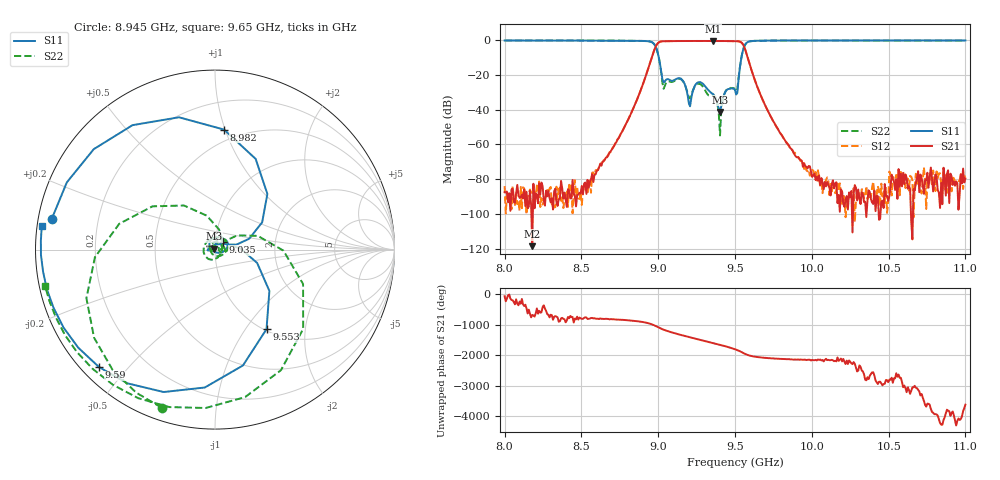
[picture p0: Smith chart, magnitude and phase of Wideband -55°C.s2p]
!Agilent Technologies,N5230C,MY49001174,A.09.42.22
!Agilent N5230C: A.09.42.22
!Date: Friday, February 13, 2026 11:53:42
!Correction: S11(Full 2 Port(1,2))
!S21(Full 2 Port(1,2))
!S12(Full 2 Port(1,2))
!S22(Full 2 Port(1,2))
!S2P File: Measurements: S11, S21, S12, S22:
# Hz S  dB  R 50
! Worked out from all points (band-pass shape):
!   401 points, 8 GHz to 11 GHz, reference 50 ohm
!   highest |S21| = -0.37 dB at 9.357 GHz (marker M1); lowest = -118.6 dB at 8.18 GHz (marker M2)
!   |S21| within 3 dB of the highest: 8.985 GHz to 9.558 GHz (572.2 MHz wide, 6.17 % of centre)
!   lowest |S11| = -41.2 dB at 9.402 GHz (marker M3), VSWR 1.02, Z = 49.3 + j0.464 ohm
!   |S11| at or under -10 dB: 9.004 GHz to 9.542 GHz (537.7 MHz wide, 5.8 % of centre)
!   |S22| runs from -54.8 to -0.1 dB; largest |S21 - S12| = 0.0016
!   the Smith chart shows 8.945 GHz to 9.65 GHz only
!   S11 on the Smith chart (normalised r, x): 8.945 GHz: 0.04, +0.09; 8.982 GHz: 0.41, +0.99; 9.035 GHz: 1.09, +0.09; 9.553 GHz: 1.02, -1.26; 9.59 GHz: 0.05, -0.42; 9.65 GHz: 0.01, +0.07
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8e9  -0.11 72.6  -87.47 -62.7  -84.00 102.4  -0.11 85.9
8.18e9  -0.11 57.3  -118.63 43.0  -87.92 134.0  -0.12 71.3
8.5025e9  -0.14 19.8  -83.91 -83.2  -94.87 -136.0  -0.14 37.7
8.8475e9  -0.28 -85.2  -37.28 -154.2  -37.32 -154.2  -0.24 -38.8
8.945e9  -0.67 169.4  -13.50 117.7  -13.50 117.7  -0.64 -108.7
8.9825e9  -3.47 85.7  -3.85 41.1  -3.85 41.2  -3.47 -176.3
9.005e9  -10.36 30.0  -1.13 -17.6  -1.12 -17.5  -10.45 125.1
9.035e9  -24.32 43.9  -0.53 -82.8  -0.53 -82.8  -27.92 -19.8
9.095e9  -23.32 53.9  -0.44 178.3  -0.44 178.3  -23.91 124.1
9.155e9  -22.67 16.7  -0.41 94.5  -0.41 94.5  -22.95 2.4
9.2375e9  -26.35 130.2  -0.38 -11.5  -0.37 -11.5  -26.65 24.2
9.2975e9  -25.62 76.3  -0.37 -86.0  -0.36 -85.9  -27.64 -63.5
9.3575e9  -30.90 85.2  -0.37 -161.4  -0.37 -161.4  -32.01 124.8
9.4025e9  -41.22 147.2  -0.38 139.7  -0.39 139.7  -54.81 -54.0
9.4475e9  -28.50 -174.8  -0.42 76.9  -0.42 76.8  -28.25 134.4
9.5e9  -28.69 171.5  -0.49 -6.7  -0.49 -6.7  -28.37 -1.3
9.5525e9  -5.55 -57.1  -2.43 -125.1  -2.43 -125.1  -5.57 -21.3
9.59e9  -0.73 -134.6  -12.15 152.6  -12.15 152.7  -0.78 -106.2
9.65e9  -0.23 172.3  -27.88 94.5  -27.89 94.6  -0.28 -168.0
1.00025e10  -0.10 84.9  -78.72 3.2  -74.66 -14.4  -0.12 90.2
1.0505e10  -0.09 38.8  -89.83 72.5  -75.60 4.3  -0.11 39.9
1.1e10  -0.09 7.3  -79.61 -30.7  -76.22 11.7  -0.12 6.9
